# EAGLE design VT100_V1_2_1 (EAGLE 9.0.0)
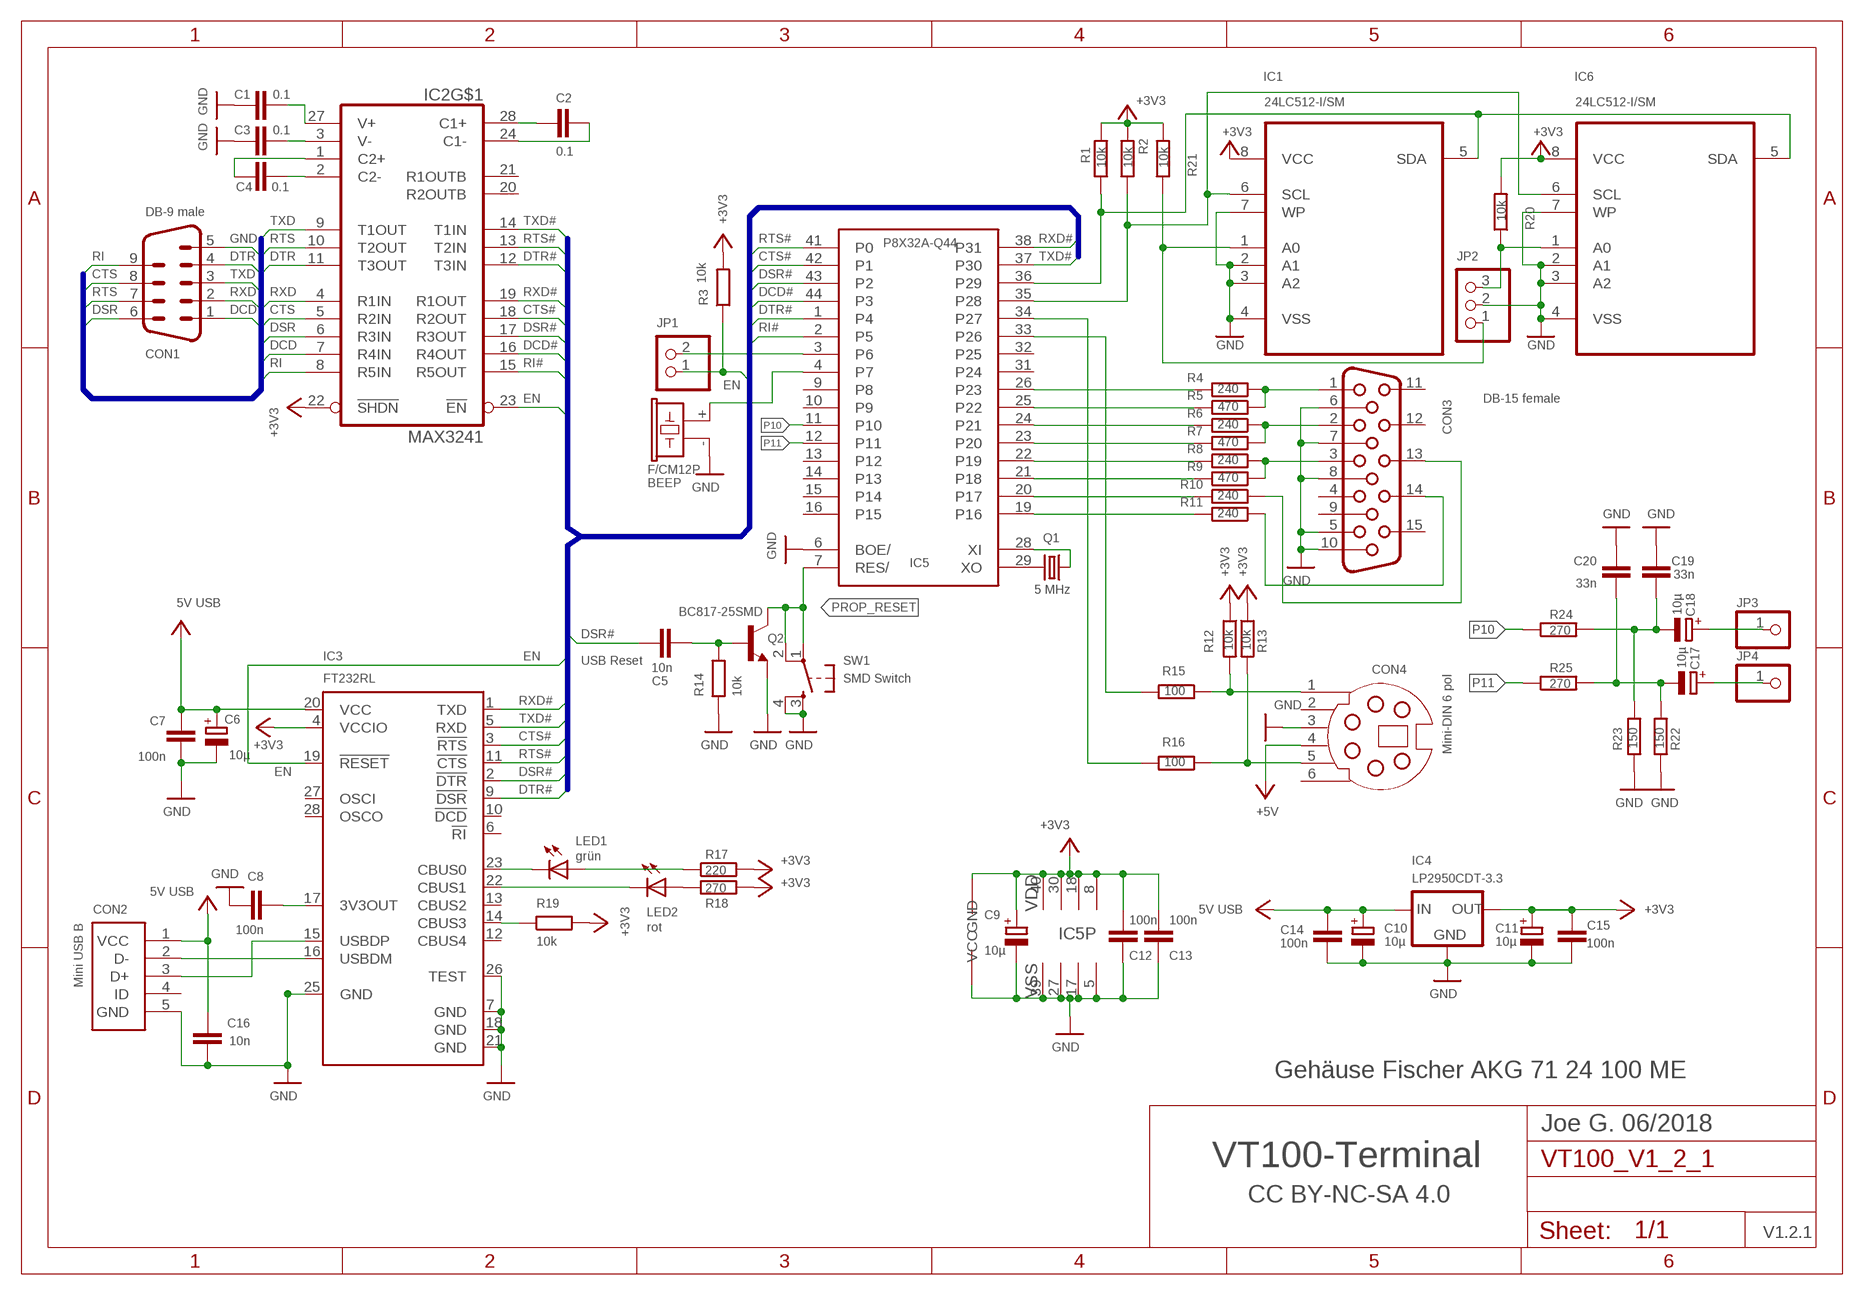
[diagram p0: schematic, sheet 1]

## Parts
BEEP  F/CM12P  [F/CM12P]
C1  0.1  C-EUC0805  [C0805]
C2  0.1  C-EUC0805  [C0805]
C3  0.1  C-EUC0805  [C0805]
C4  0.1  C-EUC0805  [C0805]
C5  10n  C-EUC0805  [C0805]
C6  10µ  CPOL-EUSMCC  [SMC_C]
C7  100n  C-EUC0805  [C0805]
C8  100n  C-EUC0805  [C0805]
C9  10µ  CPOL-EUSMCC  [SMC_C]
C10  10µ  CPOL-EUSMCC  [SMC_C]
C11  10µ  CPOL-EUSMCC  [SMC_C]
C12  100n  C-EUC0805  [C0805]
C13  100n  C-EUC0805  [C0805]
C14  100n  C-EUC0805  [C0805]
C15  100n  C-EUC0805  [C0805]
C16  10n  C-EUC0805  [C0805]
C17  10µ  CPOL-EUSMCC  [SMC_C]
C18  10µ  CPOL-EUSMCC  [SMC_C]
C19  33n  C-EUC0805  [C0805]
C20  33n  C-EUC0805  [C0805]
CON1  DB-9 male  M09-182  [182-009-MALE]
CON2  Mini USB B  65100516121  [65100516121]
CON3  DB-15 female  HF15H  [HDF15H]
CON4  Mini-DIN 6 pol  MDSSV-BC06  [SSV-BC06]
IC1  24LC512-I/SM  [SOIC127P794X203-8N]
IC2  MAX3241  [SSOP28]
IC3  FT232RL  [SSOP28]
IC4  LP2950CDT-3.3  [DPACK]
IC5  P8X32A-Q44  [P8X32A-Q44]
IC6  24LC512-I/SM  [SOIC127P794X203-8N]
JP1  PINHD-1X2  [1X02]
JP2  PINHD-1X3  [1X03]
JP3  PINHD-1X1  [1X01]
JP4  PINHD-1X1  [1X01]
LED1  grün  LEDSMT1206  [1206]
LED2  rot  LEDSMT1206  [1206]
Q1  5 MHz  CRYSTALHC49S  [HC49/S]
Q2  BC817-25SMD  [SOT23-BEC]
R1  10k  R-EU_M0805  [M0805]
R2  10k  R-EU_M0805  [M0805]
R3  10k  R-EU_M0805  [M0805]
R4  240  R-EU_R0805  [R0805]
R5  470  R-EU_R0805  [R0805]
R6  240  R-EU_R0805  [R0805]
R7  470  R-EU_R0805  [R0805]
R8  240  R-EU_R0805  [R0805]
R9  470  R-EU_R0805  [R0805]
R10  240  R-EU_R0805  [R0805]
R11  240  R-EU_M0805  [M0805]
R12  10k  R-EU_M0805  [M0805]
R13  10k  R-EU_M0805  [M0805]
R14  10k  R-EU_M0805  [M0805]
R15  100  R-EU_M0805  [M0805]
R16  100  R-EU_M0805  [M0805]
R17  220  R-EU_M0805  [M0805]
R18  270  R-EU_M0805  [M0805]
R19  10k  R-EU_M0805  [M0805]
R20  10k  R-EU_M0805  [M0805]
R21  10k  R-EU_M0805  [M0805]
R22  150  R-EU_M0805  [M0805]
R23  150  R-EU_M0805  [M0805]
R24  270  R-EU_M0805  [M0805]
R25  270  R-EU_M0805  [M0805]
SW1  SMD Switch  DTSM-6  [DTSM-6]

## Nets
+3V3: C9.+ C11.+ C12.2 C13.2 C15.2 IC1.8(VCC) IC2.22(!SHDN) IC2.26(VCC) IC3.4(VCCIO) IC4.3(OUT) IC5.8(VDD) IC5.18(VDD) IC5.30(VDD) IC5.40(VDD) IC6.8(VCC) R1.2 R2.2 R3.2 R12.1 R13.1 R17.2 R18.2 R19.2 R20.2 R21.2
+5V: C6.+ C7.2 C10.+ C14.2 C16.2 CON2.1(VCC) CON4.4 IC3.20(VCC) IC4.1(IN) ; supply symbol labelled 5V USB
CTS: CON1.8 IC2.5(R2IN)
CTS#: IC2.18(R2OUT) IC3.3(!RTS) IC5.42(P1)
DCD: CON1.1 IC2.7(R4IN)
DCD#: IC2.16(R4OUT) IC5.44(P3)
DM: CON2.2(D-) IC3.16(USBDM)
DP: CON2.3(D+) IC3.15(USBDP)
DSR: CON1.6 IC2.6(R3IN)
DSR#: C5.1 IC2.17(R3OUT) IC3.2(!DTR) IC5.43(P2)
DTR: CON1.4 IC2.11(T3OUT)
DTR#: IC2.12(T3IN) IC3.9(!DSR) IC5.1(P4)
EN: IC2.23(!EN) IC3.19(!RESET) JP1.1 R3.1
GND: BEEP.- C1.2 C3.1 C6.- C7.1 C8.1 C9.- C10.- C11.- C12.1 C13.1 C14.1 C15.1 C16.1 C19.2 C20.2 CON1.5 CON2.5(GND) CON3.5 CON3.6 CON3.7 CON3.8 CON3.10 CON4.3 IC1.2(A1) IC1.3(A2) IC1.4(VSS) IC1.7(WP) IC2.25(GND) IC3.7(GND) IC3.18(GND) IC3.21(GND) IC3.25(GND) IC3.26(TEST) IC4.4(GND) IC5.5(VSS) IC5.6(BOE/) IC5.17(VSS) IC5.27(VSS) IC5.39(VSS) IC6.2(A1) IC6.3(A2) IC6.4(VSS) IC6.7(WP) JP2.2 Q2.E R14.1 R22.2 R23.2 SW1.3 SW1.4
N$1: IC5.3(P6) JP1.2
N$2: BEEP.+ IC5.4(P7)
N$3: C4.2 IC2.2(C2-)
N$4: C5.2 Q2.B R14.2
N$5: IC5.29(XO) Q1.2
N$6: C4.1 IC2.1(C2+)
N$7: C3.2 IC2.3(V-)
N$8: IC3.23(CBUS0) LED1.C
N$9: IC3.22(CBUS1) LED2.C
N$10: LED2.A R18.1
N$11: C1.1 IC2.27(V+)
N$12: IC5.28(XI) Q1.1
N$13: C2.1 IC2.28(C1+)
N$14: C8.2 IC3.17(3V3OUT)
N$15: C2.2 IC2.24(C1-)
N$16: IC1.1(A0) JP2.1 R21.1
N$17: CON3.1 R4.1 R5.1
N$18: IC5.26(P23) R4.2
N$19: IC5.25(P22) R5.2
N$20: CON3.2 R6.1 R7.1
N$21: IC5.24(P21) R6.2
N$22: IC5.23(P20) R7.2
N$23: LED1.A R17.1
N$24: IC6.1(A0) JP2.3 R20.1
N$25: CON3.3 R8.1 R9.1
N$26: IC5.22(P19) R8.2
N$27: IC5.21(P18) R9.2
N$28: IC5.20(P17) R10.2
N$29: IC5.19(P16) R11.2
N$30: CON3.13 R10.1
N$31: CON3.14 R11.1
N$32: C17.- C20.1 R22.1 R25.2
N$33: C18.- C19.1 R23.1 R24.2
N$34: CON4.1 R12.2 R15.1
N$35: C18.+ JP3.1
N$36: CON4.5 R13.2 R16.1
N$37: C17.+ JP4.1
N$39: IC3.14(CBUS3) R19.1
P10: IC5.11(P10) R24.1
P11: IC5.12(P11) R25.1
P26: IC5.33(P26) R15.2
P27: IC5.34(P27) R16.2
PROP_RESET: IC5.7(RES/) Q2.C SW1.1 SW1.2
RI: CON1.9 IC2.8(R5IN)
RI#: IC2.15(R5OUT) IC5.2(P5)
RTS: CON1.7 IC2.10(T2OUT)
RTS#: IC2.13(T2IN) IC3.11(!CTS) IC5.41(P0)
RXD: CON1.2 IC2.4(R1IN)
RXD#: IC2.19(R1OUT) IC3.1(TXD) IC5.38(P31)
SCL: IC1.6(SCL) IC5.35(P28) IC6.6(SCL) R2.1
SDA: IC1.5(SDA) IC5.36(P29) IC6.5(SDA) R1.1
TXD: CON1.3 IC2.9(T1OUT)
TXD#: IC2.14(T1IN) IC3.5(RXD) IC5.37(P30)
Unconnected: CON2.4(ID) CON3.4 CON3.9 CON3.11 CON3.12 CON3.15 CON4.2 CON4.6 IC2.20(R2OUTB) IC2.21(R1OUTB) IC3.6(!RI) IC3.10(!DCD) IC3.12(CBUS4) IC3.13(CBUS2) IC3.27(OSCI) IC3.28(OSCO) IC5.9(P8) IC5.10(P9) IC5.13(P12) IC5.14(P13) IC5.15(P14) IC5.16(P15) IC5.31(P24) IC5.32(P25)

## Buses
DTE,DSR,DTR,RTS,CTS,TXD,RXD,RI,DCD,GND
TXD#,RXD#,RTS#,CTS#,DSR#,DCD#,DTR#,RI#,EN,DCD_U,RI_U

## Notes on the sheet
- USB Reset
- Gehäuse Fischer AKG 71 24 100 ME
- Joe G. 06/2018
- VT100-Terminal
- CC BY-NC-SA 4.0
- V1.2.1

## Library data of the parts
BEEP = buzzer:F/CM12P: BUZZER
C1-C5 C7 C8 C12-C16 C19 C20 = rcl:C-EU: CAPACITOR, European symbol
C6 C9-C11 C17 C18 = rcl:CPOL-EU: POLARIZED CAPACITOR, European symbol
CON1 = con-subd:M09: SUB-D; OC_FARNELL: unknown; OC_NEWARK: unknown
CON2 = Wuerth_Elektronik_eiCan_11_Communication_Connectors_2_4:65100516121: WR-COM SMT Horizontal 5 Contacts Mini USB Typ B
CON3 = con-subd:HF15: SUB-D; OC_FARNELL: unknown; OC_NEWARK: unknown
CON4 = con-yamaichi:MDSSV-BC06: YAMAICHI CONNECTOR; OC_FARNELL: unknown; OC_NEWARK: unknown
IC1 IC6 = 24LC512:24LC512-I/SM: 512K I2C Serial EEPROM; MPN: 24LC512-I/SM; OC_FARNELL: 9758038; OC_NEWARK: 62K0582; PACKAGE: SOIC-8; SUPPLIER: MICROCHIP
IC2 = Maxim_New:MAX3241: MAX3241
IC3 = ftdichip:FT232R: Source: http://www.ftdichip.com/Documents/DataSheets/DS_FT232R_v104.pdf
IC4 = v-reg:LP2950?*: Source: http://cache.national.com/ds/LP/LP2950.pdf
IC5 = parallax_propeller:P8X32A-Q44
JP1 = pinhead:PINHD-1X2: PIN HEADER
JP2 = pinhead:PINHD-1X3: PIN HEADER
JP3 JP4 = pinhead:PINHD-1X1: PIN HEADER
LED1 LED2 = led:LED: LED
Q1 = crystal:CRYSTAL: CRYSTAL; OC_FARNELL: 1667008; OC_NEWARK: unknown
Q2 = transistor-npn:BC817*: NPN Transistor
R1-R25 = rcl:R-EU_: RESISTOR, European symbol
SW1 = switch-tact:DTSM-6

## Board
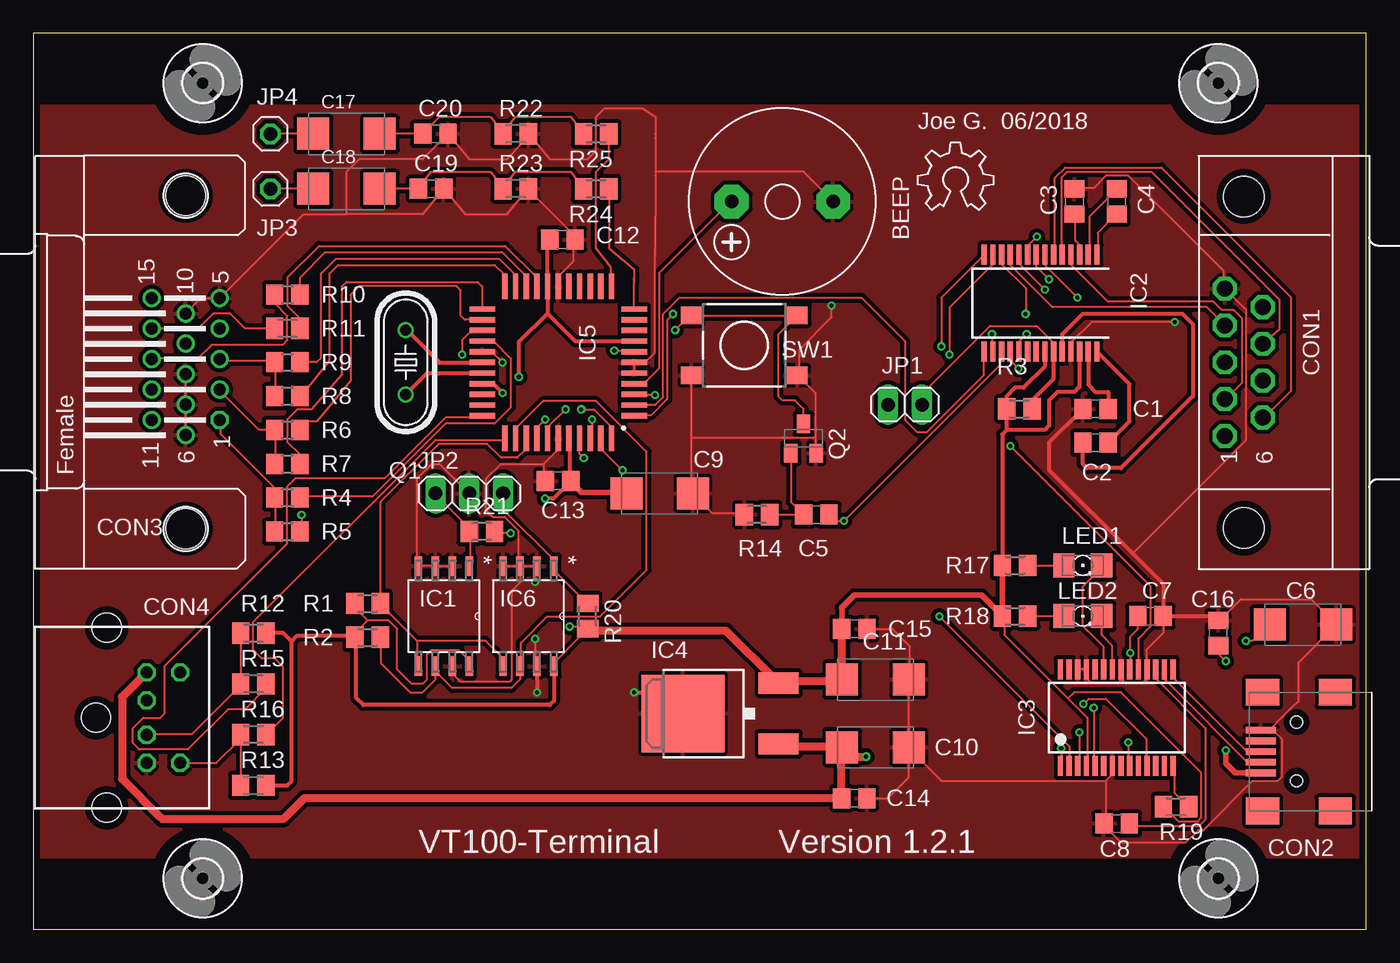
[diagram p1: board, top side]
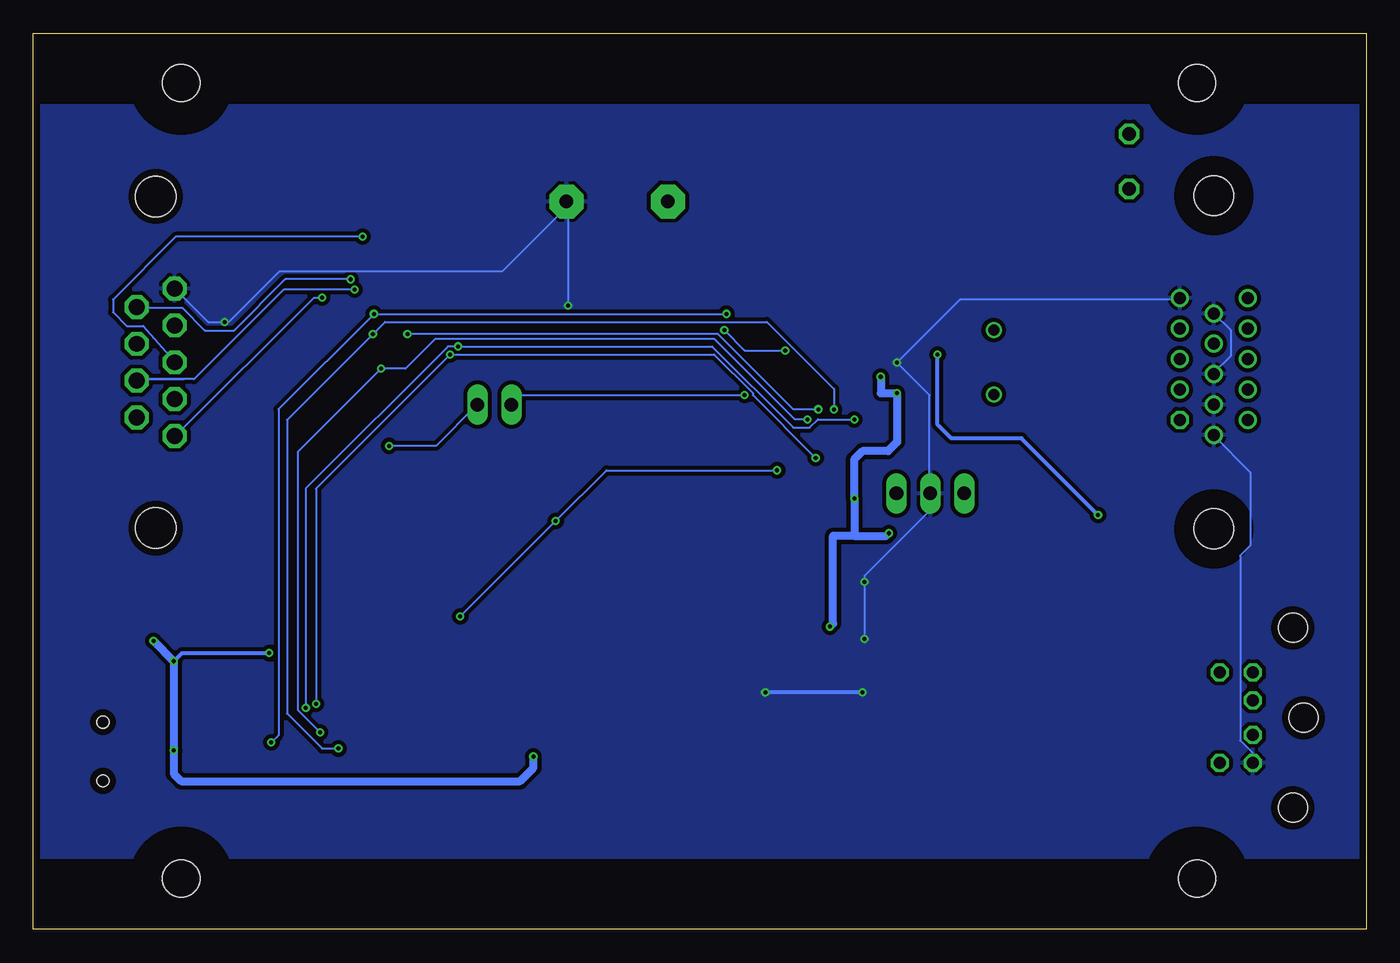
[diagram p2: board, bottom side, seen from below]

Size 100 x 67.23 mm. Coordinates in mm from the lower left corner, seen from the top.
Outline: 0,0 100,0 100,67.23 0,67.23 0,0
Copper layers (1*16): Top 0.035mm / dielectric 1.6mm / Bottom 0.035mm
Design rules "Elecrow_2-layer_PCB_eagle_rule": minimum track width 6mil, minimum drill 12mil, track to track 6mil, track to pad 6mil, pad to pad 6mil, via to via 8mil, smd to smd 0mil, copper to edge 20mil, drill to drill 10mil, minimum pad ring 6mil, minimum via ring 6mil, stop-mask expansion 0mil, vias tented up to drill 100mil, thermal gap 10mil
tRestrict: area 0,0 to 100,5; area 0,62.2 to 100,67.2
bRestrict: area 0,62.2 to 100,67.2; area 0,0 to 100,5

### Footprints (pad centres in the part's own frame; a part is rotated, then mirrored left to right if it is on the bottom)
F/CM12P = drill 1.016 pad 2.54 octagon: + 3.81,0; - -3.81,0
C0805 = smd 1.3 x 1.5: 1 -0.95,0; 2 0.95,0
SMC_C = smd 2.4 x 2.4: + -2.5,0; - 2.5,0
182-009-MALE = drill 1.194 pad 1.524 octagon: 1 -5.537,10.923; 2 -2.769,10.923; 3 0,10.923; 4 2.769,10.923; 5 5.537,10.923; 6 -4.153,8.08; 7 -1.384,8.08; 8 1.384,8.08; 9 4.153,8.08 | hole 3.048: -12.446,9.501; 12.446,9.501
65100516121 = smd 0.5 x 2.25: 1 -1.6,5.685; 2 -0.8,5.685; 3 0,5.685; 4 0.8,5.685; 5 1.6,5.685 | smd 2 x 2.5: Z1 -4.45,5.56; Z2 4.45,5.56; Z3 4.45,0.11; Z4 -4.45,0.11 | hole 0.9: -2.2,3.01; 2.2,3.01
HDF15H = drill 0.9 octagon: 1 4.329,2.54 | drill 0.9: 2 2.043,2.54; 3 -0.243,2.54; 4 -2.529,2.54; 5 -4.815,2.54; 6 5.472,0; 7 3.186,0; 8 0.9,0; 9 -1.386,0; 10 -3.672,0; 11 4.329,-2.54; 12 2.043,-2.54; 13 -0.243,-2.54; 14 -2.529,-2.54; 15 -4.815,-2.54 | hole 3: -12.5,0; 12.5,0
SSV-BC06 = drill 0.9 octagon: 1 1.3,8.5; 2 -1.3,8.5; 3 3.4,8.5; 4 -3.4,8.5; 5 3.4,11; 6 -3.4,11 | hole 2.2: -6.75,5.5; 0,4.7; 6.75,5.5
SOIC127P794X203-8N = smd 1.473 x 0.559: 1 -3.759,1.905; 2 -3.759,0.635; 3 -3.759,-0.635; 4 -3.759,-1.905; 5 3.759,-1.905; 6 3.759,-0.635; 7 3.759,0.635; 8 3.759,1.905
SSOP28 = smd 0.4 x 1.5: 1 -4.225,-3.625; 2 -3.575,-3.625; 3 -2.925,-3.625; 4 -2.275,-3.625; 5 -1.625,-3.625; 6 -0.975,-3.625; 7 -0.325,-3.625; 8 0.325,-3.625; 9 0.975,-3.625; 10 1.625,-3.625; 11 2.275,-3.625; 12 2.925,-3.625; 13 3.575,-3.625; 14 4.225,-3.625; 15 4.225,3.625; 16 3.575,3.625; 17 2.925,3.625; 18 2.275,3.625; 19 1.625,3.625; 20 0.975,3.625; 21 0.325,3.625; 22 -0.325,3.625; 23 -0.975,3.625; 24 -1.625,3.625; 25 -2.275,3.625; 26 -2.925,3.625; 27 -3.575,3.625; 28 -4.225,3.625
DPACK = smd 1.6 x 3: 1 -2.28,-4.8; 3 2.28,-4.8 | smd 5.8 x 6.2: 4 0,2.38
P8X32A-Q44 = smd 1.9 x 0.4: 1 -5.713,4.013; 2 -5.713,3.212; 3 -5.713,2.413; 4 -5.713,1.613; 5 -5.713,0.812; 6 -5.713,0.013; 7 -5.713,-0.787; 8 -5.713,-1.587; 9 -5.713,-2.388; 10 -5.713,-3.188; 11 -5.713,-3.987; 23 5.688,-3.987; 24 5.688,-3.188; 25 5.688,-2.388; 26 5.688,-1.587; 27 5.688,-0.787; 28 5.688,0.013; 29 5.688,0.812; 30 5.688,1.613; 31 5.688,2.413; 32 5.688,3.212; 33 5.688,4.013 | smd 0.4 x 1.9: 12 -4.013,-5.688; 13 -3.212,-5.688; 14 -2.413,-5.688; 15 -1.613,-5.688; 16 -0.812,-5.688; 17 -0.013,-5.688; 18 0.787,-5.688; 19 1.587,-5.688; 20 2.388,-5.688; 21 3.188,-5.688; 22 3.987,-5.688; 34 3.987,5.713; 35 3.188,5.713; 36 2.388,5.713; 37 1.587,5.713; 38 0.787,5.713; 39 -0.013,5.713; 40 -0.812,5.713; 41 -1.613,5.713; 42 -2.413,5.713; 43 -3.212,5.713; 44 -4.013,5.713
1X02 = drill 1.016 long: 1 -1.27,0; 2 1.27,0
1X03 = drill 1.016 long: 1 -2.54,0; 2 0,0; 3 2.54,0
1X01 = drill 1.016 octagon: 1 0,0
1206 = smd 1.6 x 1.803: A -1.422,0; C 1.422,0
HC49/S = drill 0.813: 1 -2.413,0; 2 2.413,0
SOT23-BEC = smd 1 x 1.4: B -0.95,-1.1; C 0,1.1; E 0.95,-1.1
M0805 = smd 1.3 x 1.6: 1 -0.95,0; 2 0.95,0
R0805 = smd 1.3 x 1.5: 1 -0.95,0; 2 0.95,0
DTSM-6 = smd 1.55 x 1.3: 1 -3.975,2.25; 2 3.975,2.25; 3 -3.975,-2.25; 4 3.975,-2.25
2,8 = hole 2.8: 0,0

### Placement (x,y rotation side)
BEEP  56.2,54.61 180 top
C1  79.69,39.05 180 top
C2  79.69,36.51 180 top
C3  78.11,54.61 270 top
C4  81.28,54.61 90 top
C5  58.74,31.11 180 top
C6  95.25,22.86 0 top
C7  83.82,23.5 180 top
C8  81.28,7.94 0 top
C9  46.99,32.7 0 top
C10  63.18,13.65 0 top
C11  63.18,18.73 0 top
C12  39.69,51.75 180 top
C13  39.37,33.66 0 top
C14  61.59,9.84 180 top
C15  61.59,22.54 180 top
C16  88.9,22.23 270 top
C17  23.5,59.69 0 top
C18  23.5,55.56 0 top
C19  29.84,55.56 0 top
C20  30.16,59.69 0 top
CON1  100.33,42.55 90 top
CON2  97.79,13.34 90 top
CON3  11.43,42.55 270 top
CON4  0,15.88 270 top
IC1  30.8,23.5 270 top
IC2  75.56,46.99 180 top
IC3  81.28,15.88 0 top
IC4  51.12,16.19 90 top
IC5  39.37,42.55 180 top
IC6  37.15,23.5 270 top
JP1  65.41,39.37 180 top
JP2  32.7,32.7 0 top
JP3  17.78,55.56 0 top
JP4  17.78,59.69 0 top
LED1  78.74,27.3 0 top
LED2  78.74,23.5 0 top
Q1  27.94,42.55 270 top
Q2  57.78,36.83 0 top
R1  25.08,24.45 180 top
R2  25.08,21.91 180 top
R3  73.98,39.05 180 top
R4  19.05,32.38 0 top
R5  19.05,29.84 0 top
R6  19.05,37.47 0 top
R7  19.05,34.92 0 top
R8  19.05,40.01 0 top
R9  19.05,42.55 0 top
R10  19.05,47.62 0 top
R11  19.05,45.09 0 top
R12  16.51,22.23 180 top
R13  16.51,10.79 180 top
R14  54.29,31.11 0 top
R15  16.51,18.41 0 top
R16  16.51,14.61 0 top
R17  73.66,27.3 180 top
R18  73.66,23.5 180 top
R19  85.72,9.21 180 top
R20  41.59,23.5 270 top
R21  33.66,29.84 0 top
R22  36.2,59.69 0 top
R23  36.2,55.56 0 top
R24  42.23,55.56 180 top
R25  42.23,59.69 180 top
SW1  53.34,43.81 0 top
U$1  [2,8]  12.7,63.5 0 top
U$3  [OSHW_6X200_NOTEXT]  66.36,53.98 0 top
U$4  [2,8]  88.9,63.5 0 top
U$5  [2,8]  88.9,3.81 0 top
U$6  [2,8]  12.7,3.81 0 top

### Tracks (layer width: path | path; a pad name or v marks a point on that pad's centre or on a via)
+3V3  (via drill 0.3)
  Top 0.152: C12.2 38.71,51.66 38.58,51.54 | 38.71,47.36 IC5.18 38.71,48.16 38.71,48.35 | 40.23,33.68 C13.2 | 40.23,36.73 IC5.40 | v35.81,29.72 34.75,29.72 R21.2 | 40.23,33.53 C13.2 | 34.59,40.84 33.83,40.84 IC5.30 | 44.35,32.77 C9.+ | 40.39,33.53 C13.2 | 17.53,10.82 R13.1 | 17.53,22.1 R12.1 | R2.2 24.23,21.95 24.32,22.04 24.32,22.42 25.08,23.18 | 24.23,24.08 24.23,24.38 R1.2 24.13,24.13 25.08,23.18 | 24.08,21.79 R2.2 | 41.45,22.4 41,21.95 | 41.45,22.4 R20.2 | 60.66,22.4 C15.2 60.66,22.55 | 60.66,18.75 C11.+ 60.66,18.59 | 55.93,18.59 IC4.3 55.78,18.59 | R20.2 41.6,22.4 41.45,22.4 | 78.49,42.67 78.49,43.28 IC2.26 | 77.64,17.31 72.85,22.1 72.85,23.47 R18.2 | 77.64,17.31 79.1,15.85 79.1,12.34 IC3.4 | 72.69,27.28 R17.2 72.69,27.43 | 72.69,23.62 R18.2 | R19.2 84.89,9.14 85.95,8.08 87.33,8.08 87.63,8.38 87.63,11.75 81.6,17.78 78.11,17.78 77.64,17.31 | 72.69,24.4 R18.2 | 24.23,21.79 R2.2 | 39.17,19.66 IC6.8 39.17,19.85 39.17,20.12 41,21.95 | 41,21.95 R20.2 | IC1.8 32.63,19.81 32.61,19.81 32.61,20.25 31.91,20.95 29.84,20.95 29.53,20.64 29.53,18.73 29.21,18.41 28.39,18.41 27.3,19.5 27.3,22.54 26.67,23.18 25.08,23.18 | v40.23,22.71 41.6,22.71 41.91,22.4 | 78.49,40.71 78.42,40.64 | 60.64,24.13 60.66,24.12
  Top 0.305: 40.23,36.73 40.23,33.68 | v38.41,32.31 39.01,32.31 40.23,33.53 | v35.2,40.23 34.59,40.84 | 72.69,27.43 72.69,37.13 73.03,37.47 | IC6.8 39.05,17.14 38.73,16.83 24.77,16.83 24.23,17.36 24.23,21.79 | R13.1 19.05,10.79 19.37,11.11 19.37,21.59 | 19.37,21.59 18.73,22.22 R12.1 | 19.37,21.59 19.81,22.04 24.32,22.04 | v36.42,41.45 36.42,44.04 38.58,46.2 | 78.42,40.64 78.11,40.32 76.83,40.32 76.2,39.69 76.2,37.78 75.88,37.47 73.03,37.47 | IC2.22 75.89,42.87 75.88,42.86 75.88,42.23 74.3,40.64 73.66,40.64 73.03,40.01 R3.2 73.03,37.47 | 38.58,51.54 IC5.18 38.58,46.2 | 38.58,46.2 40.65,44.13 IC5.8 | IC2.26 78.49,40.71
  Top 0.406: 44.35,32.77 41.15,32.77 40.39,33.53 | 72.69,23.62 72.69,24.4 72.69,27.28 | R18.2 71.12,25.09 61.6,25.09 60.64,24.13 | 60.66,24.12 60.66,22.4
  Top 0.61: 60.66,18.75 60.66,22.4 | 60.66,18.59 55.93,18.59 | 41.6,22.4 41.91,22.4 51.97,22.4 55.78,18.59
  Bottom 0.61: v36.42,41.45 36.42,40.23 v35.2,40.23 35.2,36.55 35.88,35.88 37.78,35.88 38.42,35.24 38.42,32.32 v38.41,32.31 38.41,29.54 38.42,29.53 | v40.23,22.71 40.01,22.94 40.01,29.53 38.42,29.53 | 38.42,29.53 36.01,29.53 v35.81,29.72
+5V  (via drill 0.3)
  Top 0.152: IC3.20 82.3,19.51 v82.3,20.73 82.3,21.97 82.87,22.55 C7.2 82.75,23.47 | v90.98,21.64 91.44,21.64 92.66,22.86 C6.+ | 89,21.18 C16.2 88.9,20.68 v89.46,20.12 | 90.98,11.89 92.05,11.89 CON2.1 | 60.5,9.91 C14.2 | 56.08,13.72 55.93,13.87 IC4.1 | 60.66,13.72 C10.+ 60.81,13.56 61,13.37 61.42,12.95 | 9.68,8.26 9.53,8.41
  Top 0.406: CON2.1 92.09,11.75 90.17,11.75 89.46,12.46 v89.46,13.41
  Top 0.61: 56.08,13.72 60.66,13.72 | 61.42,12.95 v62.48,12.95 | 61,13.37 60.65,13.02 C14.2 20.32,9.84 18.73,8.26 9.68,8.26 | CON4.4 6.67,17.44 6.67,11.27 9.53,8.41
  Bottom 0.305: v82.3,20.73 88.85,20.73 v89.46,20.12
  Bottom 0.61: v90.98,21.64 v89.46,20.12 v89.46,13.41 89.46,11.67 88.9,11.11 63.5,11.11 62.48,12.13 v62.48,12.95
CTS
  Top 0.152: IC2.5 77.11,50.75 77.11,56.39 77.57,56.84 83.88,56.84 93.47,47.26 93.47,45 CON1.8
CTS#  (via drill 0.3)
  Top 0.152: v78.49,14.78 78.49,12.34 IC3.3 | v73.91,42.06 73.3,42.67 73.3,43.28 IC2.18 | v41.91,38.25 41.91,36.88 IC5.42
  Bottom 0.152: v78.49,14.78 80.16,16.46 80.16,35.81 v73.91,42.06 | 73.76,42.06 v73.91,42.06 | v41.91,38.25 42.86,38.25 48.88,44.27 69.87,44.27 72.08,42.06 v73.91,42.06
DCD  (via drill 0.3)
  Top 0.152: v78.33,47.4 75.89,49.84 75.89,50.6 IC2.7
  Bottom 0.152: v78.33,47.4 78.94,47.4 89.31,37.03 CON1.1
DCD#  (via drill 0.3)
  Top 0.152: v71.93,44.65 71.93,43.43 IC2.16 | IC5.44 43.38,37.69 42.06,39.01 v41.11,39.01
  Bottom 0.152: v71.93,44.65 48.62,44.65 42.98,39.01 v41.11,39.01
DM
  Top 0.152: IC3.16 84.89,19.36 84.89,18.75 85.63,18 90.98,12.65 92.05,12.65 CON2.2
DP
  Top 0.152: IC3.15 85.65,19.36 85.65,18.75 90.98,13.41 92.05,13.41 CON2.3
DSR
  Top 0.152: IC2.6 76.66,50.75 76.66,56.39 77.42,57.15 84.63,57.15 94.37,47.41 94.37,40.42 92.99,39.04 CON1.6
DSR#  (via drill 0.3)
  Top 0.152: v67.97,23.47 77.72,13.72 77.72,12.34 IC3.2 | C5.1 59.74,31.09 60.2,30.63 v60.81,30.63 72.54,42.37 72.54,43.28 IC2.17 | v44.2,34.44 42.67,35.97 42.67,36.73 IC5.43
  Bottom 0.152: v67.97,23.47 v60.81,30.63 57,34.44 v44.2,34.44
DTR
  Top 0.152: IC2.11 73.3,50.6 73.3,49.84 76.33,46.81 76.35,46.79 76.47,46.67 88.05,46.67 CON1.4
DTR#  (via drill 0.3)
  Top 0.152: v82.14,14.02 82.14,12.34 IC3.9 | 72.69,49.84 72.69,50.6 IC2.12 72.64,49.91 74.45,48.1 v74.45,46.18 | v48.01,46.18 47.55,45.72 47.55,39.78 46.33,38.56 45.11,38.56 IC5.1
  Bottom 0.152: v48.01,46.18 v74.45,46.18 81.6,39.03 81.6,14.57 v82.14,14.02
EN  (via drill 0.3)
  Top 0.152: 76.5,42.67 76.5,43.28 IC2.23 76.5,43.43 76.5,44.04 75.29,45.26 71.78,45.26 66.75,40.23 66.75,39.47 JP1.1 | v73.3,36.27 83.82,25.76 83.82,22.71 82.91,21.79 IC3.19
  Top 0.305: IC2.23 76.52,43.34 76.52,41.27 74.93,39.69 R3.1
  Bottom 0.152: v73.3,36.27 69.8,36.27 66.75,39.32 JP1.1
GND  (via drill 0.3)
  Top 0.152: 65.53,18.75 C11.- | 80.47,11.12 80.47,8.08 C8.1 | 80.47,11.12 80.92,11.58 80.92,12.19 IC3.7 | 62.64,9.91 C14.1 64.14,9.84 65.68,11.39 65.68,13.72 | 65.53,13.56 C10.- | 80.47,11.12 68.12,11.12 65.68,13.56 C10.- | 65.68,13.72 65.68,18.59 C11.- | 65.68,13.72 C10.- | 50.9,16.15 48.77,16.15 IC4.4 | v85.65,45.57 79.4,45.57 77.88,44.04 77.88,43.43 IC2.25 | C3.1 78.18,55.63 79.55,55.63 80.47,56.54 82.14,56.54 89.31,49.38 89.31,48.16 CON1.5 | IC3.26 78.49,19.51 78.94,19.51 IC3.25 79.1,19.36 79.1,18.75 79.4,18.44 81.38,18.44 81.69,18.75 | 81.69,18.75 81.69,19.36 IC3.21 | 81.69,18.75 81.99,18.44 83.21,18.44 83.52,18.75 83.52,19.36 IC3.18 | 84.89,23.47 85.04,23.47 C7.1 | 88.7,23.47 88.85,23.32 C16.1 89,23.16 90.6,24.77 95.89,24.77 97.75,22.9 C6.- 94.93,20.04 94.93,17.14 94.36,16.57 94.35,16.57 93.75,15.96 92.72,14.94 CON2.5 | 84.89,23.47 C7.1 | 92.05,14.94 CON2.5 | 83.67,19.51 IC3.18 | 89.46,48.01 CON1.5 | 80.47,7.92 C8.1 | 92.2,14.78 CON2.5 | 58.67,36.88 58.67,40.23 57.45,41.45 SW1.4 | 58.67,36.88 58.67,35.81 Q2.E | 49.38,36.88 49.38,32.77 C9.- 49.53,32.61 50.9,31.24 53.34,31.24 R14.1 | 49.38,36.88 49.38,41.45 SW1.3 | 49.38,36.88 58.67,36.88 | 45.11,41.76 IC5.5 IC5.6 | 45.11,42.52 IC5.6 | 46.63,50.48 46.63,43.28 45.88,42.53 IC5.6 | 46.63,50.48 46.63,51.05 | 59.05,55.56 59.89,54.71 BEEP.- | 59.05,55.56 58.37,56.24 | 57.45,41.6 SW1.4 | 38.28,34.92 39.32,35.97 39.32,36.73 IC5.39 | 38.56,33.68 C13.1 38.28,33.8 38.28,34.92 | IC1.7 31.55,19.66 31.55,19.09 32.07,18.57 35.72,18.57 35.88,18.73 35.88,25.4 36.51,26.04 IC6.3 | 35.36,27.13 IC6.4 IC6.3 | 36.42,27.13 IC6.3 | IC6.3 36.58,27.28 37.64,27.28 IC6.2 37.64,27.13 v37.64,26.06
  Top 0.152: IC6.3 36.42,27.28 36.42,29.87 35.36,30.94 34.47,30.94 33.97,31.43 33.97,33.81 35.09,34.92 38.28,34.92 | 28.96,27.28 30.02,27.28 IC1.3 30.18,27.28 31.39,27.28 IC1.2 | 28.8,27.28 28.96,27.28 | 28.96,27.28 IC1.4 28.8,27.28 | v37.64,21.79 37.64,19.81 IC6.7 | v35.2,42.52 34.44,43.28 33.83,43.28 IC5.27 | 28.8,27.28 28.8,33.83 29.9,34.92 30.48,34.92 30.48,34.9 32.61,32.77 JP2.2 | 31.24,59.59 C20.2 | 37.03,59.59 R22.2 | IC5.17 39.47,48.31 39.47,49.07 40.54,50.14 40.54,51.66 C12.1 40.54,51.82 40.54,52.12 37.19,55.47 R23.2 | 30.94,55.47 C19.2 | C19.2 | 37.03,55.47 R23.2 | 31.09,59.59 C20.2 | 30.79,55.47 C19.2 | 13.87,47.24 CON3.5 | CON3.6 CON3.7 CON3.8 | 14.02,47.4 CON3.5 | R22.2 37.19,59.59 35.56,57.78 32.7,57.78 C20.2 | CON1.5 90.98,46.51 90.98,36.69 82.48,28.19 | 84.77,23.58 84.89,23.47 | CON3.5 20.27,53.66 23.5,53.66 | 30.8,55.4 C19.2 | 23.5,53.66 23.5,56.83 24.45,57.78 29.21,57.78 C20.2 | 31.11,59.37 C20.2 | SW1.4 57.47,41.72 57.47,43.5 59.89,45.92 v59.89,46.79 | CON3.10 12.57,47.36 CON3.5 | CON2.5 93.02,14.94 93.66,14.29 93.66,11.43 93.36,11.12 91.45,11.12 87.77,7.44 87.39,7.44 86.46,6.51 81.6,6.51 80.33,7.78 C8.1 | 62.55,21.87 C15.1 64.45,22.54 65.72,21.27 65.72,18.77 C11.- | C7.1 84.77,22.22 83.5,20.95 83.5,19.55 IC3.18 | C19.2 32.38,53.66 35.56,53.66 R23.2 | C19.2 29.21,53.66 23.5,53.66 | 59.05,55.56 57.78,56.83 46.67,56.83 46.67,56.52 | 46.67,56.52 46.63,50.48 | 46.67,59.69 46.67,59.37 | 46.67,59.37 46.67,56.52 | R22.2 38.73,57.78 41.59,57.78 42.23,58.42 42.23,60.96 42.86,61.59 45.72,61.59 46.67,60.96 46.67,59.37
  Top 0.305: 88.7,23.47 85.04,23.47 | IC6.7 v37.78,17.78 | v45.09,17.78 46.04,17.78 48.77,16.15 | C1.2 76.2,36.51 76.2,34.47 82.48,28.19 84.77,25.89 84.77,23.58
  Bottom 0.152: CON1.5 89.31,48.01 86.87,45.57 v85.65,45.57 85.34,45.57 81.53,49.38 64.81,49.38 59.89,54.29 | 59.89,54.29 59.89,54.56 BEEP.- | 59.89,54.29 v59.89,46.79 | v37.64,21.79 v37.64,26.06 37.64,26.52 32.77,31.39 32.77,32.61 JP2.2 32.77,32.77 32.77,40.08 v35.2,42.52 30.48,47.24 14.02,47.24 CON3.5 | CON4.3 8.53,12.5 8.53,13.26 9.45,14.17 9.45,28.04 8.69,28.8 8.69,34.29 11.43,37.03 CON3.6 | CON3.8 11.43,41.76 10.16,43.03 | CON3.10 10.16,44.95 10.16,43.03 | 10.16,43.03 10.16,43.02
  Bottom 0.305: v37.78,17.78 v45.09,17.78
  pour Top (isolate 0.305): 0,67.31 100.01,67.31 100.01,0 0,0
  pour Bottom (isolate 0.305): 0,66.99 100.01,66.99 100.01,0 0,0
N$1  (via drill 0.3)
  Top 0.152: v46.63,40.08 45.11,40.08 IC5.3
  Bottom 0.152: v46.63,40.08 63.4,40.08 64.01,39.47 JP1.2
N$2
  Top 0.152: IC5.4 45.11,41 45.87,41 46.94,42.06 46.94,49.23 52.27,54.56 BEEP.+
N$3
  Top 0.152: IC2.2 79.25,50.75 79.25,53.49 81.23,55.47 C4.2
N$4
  Top 0.152: 56.84,35.66 Q2.B 56.84,32.07 C5.2 | 55.32,31.24 R14.2 C5.2 | C5.2
N$5
  Top 0.152: 33.68,41.6 IC5.29
  Top 0.305: Q1.2 29.54,41.73 IC5.29
N$6
  Top 0.152: IC2.1 79.86,50.75 79.86,52.27 81.23,53.65 C4.1
N$7
  Top 0.152: C3.2 78.18,53.65 78.18,51.66 78.49,51.36 78.49,50.75 IC2.3
N$8
  Top 0.152: LED1.C 80.01,27.28 80.01,26.99 78.74,25.72 78.74,22.76 79.1,22.4 79.17,22.33 80.31,21.19 IC3.23
N$9
  Top 0.152: 80.92,19.51 IC3.22 80.95,21.28 80.16,22.07 LED2.C | 80.16,23.47 LED2.C | LED2.C
N$10
  Top 0.152: R18.1 74.68,23.47 77.27,23.47 LED2.A
N$11
  Top 0.305: IC2.27 79.14,40.88 79.69,40.32 80.64,40.32 C1.1
N$12
  Top 0.152: IC5.28 | 28.04,44.96 Q1.1
  Top 0.305: IC5.28 30.48,42.52 28.04,44.96
N$13
  Top 0.152: 79.86,43.28 IC2.28
  Top 0.305: C2.1 82.23,38.1 82.23,40.91 79.86,43.28
N$14
  Top 0.152: 82.3,7.92 C8.2 82.39,7.77 87.48,7.77 87.94,8.23 87.94,15.09 84.28,18.75 84.28,19.36 IC3.17
N$15
  Top 0.152: 77.27,43.43 IC2.24
  Top 0.305: C2.2 78.74,34.92 79.06,34.61 81.6,34.61 86.26,39.27 87,40.01 87,45.4 86.2,46.2 78.74,46.2 77.19,44.65 IC2.24
N$16
  Top 0.152: IC1.1 32.77,27.28 32.77,29.72 R21.1 32.61,29.87 32.61,30.18 30.18,32.61 JP2.1
N$17
  Top 0.152: R5.1 18.14,29.87 18.14,32.31 R4.1 17.98,32.46 17.98,33.22 14.02,37.19 14.02,38.1 CON3.1
N$18
  Top 0.152: R4.2 20.12,32.46 25.45,32.46 30.94,37.95 34.59,37.95 35.81,39.17 35.81,42.82 34.59,44.04 33.83,44.04 IC5.26
N$19  (via drill 0.3)
  Top 0.152: v20.12,31.09 20.12,29.87 R5.2 | v32.16,43.13 32.16,44.2 32.77,44.81 33.68,44.81 IC5.25
  Bottom 0.305: v20.12,31.09 25.86,36.83 31.11,36.83 32.16,37.87 v32.16,43.13
N$20
  Top 0.152: R7.1 18.14,35.05 18.14,37.34 R6.1 17.98,37.49 16.92,37.49 14.02,40.39 CON3.2
N$21
  Top 0.152: R6.2 20.12,37.49 20.12,37.8 20.42,38.1 21.27,38.1 23.8,41.16 23.8,47.61 24.45,48.26 31.75,48.26 32.07,47.94 32.07,46.04 32.37,45.73 IC5.24
N$22
  Top 0.152: R7.2 19.96,35.05 19.96,35.66 19.05,36.58 19.05,38.25 19.81,39.01 20.88,39.01 23.18,41.63 23.18,48.26 23.5,48.58 33.34,48.58 33.68,48.23 IC5.23 33.68,46.48
N$23
  Top 0.152: R17.1 74.68,27.28 77.27,27.28 LED1.A
N$24
  Top 0.152: R20.1 41.45,24.54 39.17,26.82 39.17,27.13 IC6.1 39.01,27.28 39.01,27.74 35.36,31.39 35.36,32.61 JP2.3
N$25
  Top 0.152: R8.1 18.14,40.08 18.14,42.52 R9.1 17.98,42.67 14.02,42.67 CON3.3
N$26
  Top 0.152: 22.15,42.62 22.14,42.61 | 22.14,42.61 20.12,40.08 R8.2 | 22.14,42.61 22.23,42.7 22.23,49.21 22.86,49.85 34.61,49.85 35.38,49.07 IC5.22
N$27
  Top 0.152: 36.12,49.07 36.12,48.31 36.17,48.24 | 36.17,48.24 IC5.21 | R9.2 21.27,42.55 21.59,42.86 21.59,49.21 22.7,50.32 34.92,50.32 36.17,49.08 36.17,48.24
N$28
  Top 0.152: R10.2 20.12,47.7 | R10.2 20,48.89 21.91,50.8 35.15,50.8 36.88,49.07 36.88,48.31 IC5.20 | 19.68,48.12 19.68,47.94 R10.2
N$29
  Top 0.152: 37.64,49.05 37.64,49.07 | R11.2 19.96,45.11 19.96,45.87 19.05,46.79 19.05,48.9 21.43,51.28 35.41,51.28 37.64,49.05 | IC5.19 37.64,49.05
N$30
  Top 0.152: R10.1 18.14,47.55 18.14,46.94 19.05,46.02 19.05,44.2 18.7,43.85 13.37,43.85 12.34,42.82 8.99,42.82 CON3.13
N$31
  Top 0.152: 17.98,45.11 R11.1 15.88,45.09 14.76,46.2 13.49,46.2 12.38,45.09 8.9,45.09 | 8.9,45.09 CON3.14 | CON3.14 8.9,45.09
N$32
  Top 0.152: C20.1 29.11,59.74 26.06,59.74 C17.- | 35.36,59.74 R22.1 | 41.15,59.74 R25.2 | R25.2 | 29.26,59.74 C20.1 | R22.1 35.2,59.74 34.29,60.96 30.48,60.96 C20.1 | R22.1 36.2,60.96 40.32,60.96 R25.2
N$33
  Top 0.152: C19.1 28.8,55.63 26.06,55.63 C18.- | 35.36,55.63 R23.1 | 41.15,55.63 R24.2 40.32,56.83 36.2,56.83 R23.1 | 28.96,55.63 C19.1 | R23.1 35.2,55.63 34.29,56.83 29.84,56.83 C19.1
N$34
  Top 0.152: R12.2 15.54,22.1 15.54,18.44 R15.1 15.54,18.29 11.89,14.63 8.53,14.63 CON4.1
N$35
  Top 0.152: C18.+ 20.88,55.63 17.83,55.63 JP3.1
N$36
  Top 0.152: 15.54,14.29 15.54,14.48 R16.1 | 15.54,14.29 15.54,10.82 R13.2 | CON4.5 13.73,12.47 15.54,14.29
N$37
  Top 0.152: C17.+ 20.88,59.74 17.83,59.74 JP4.1
N$39
  Top 0.152: IC3.14 85.65,12.19 85.65,10.21 86.56,9.3 R19.1
P10
  Top 0.152: 43.28,55.47 R24.1 | R24.1 | R24.1 43.18,51.12 45.09,49.53 45.09,48.58 | IC5.11 45.09,48.58 | 45.09,48.58 45.09,48.9
P11
  Top 0.152: 43.13,59.59 R25.1 43.18,57.78 42.23,56.83 42.23,51.12 43.34,49.69 IC5.12 43.28,48.31
P26
  Top 0.152: 17.37,18.29 R15.2 17.46,18.09 15.88,16.51 14.61,16.51 11.59,13.49 7.94,13.49 7.46,13.97 7.46,15.08 8.26,15.88 9.53,15.88 9.84,16.19 9.84,19.75 19.05,28.96 19.05,33.22 19.66,33.83 26.36,33.83 30.94,38.41 33.68,38.41 IC5.33
P27
  Top 0.152: 17.53,14.63 R16.2 18.73,15.88 18.73,19.68 18.1,20.32 17.14,20.32 16.51,20.95 16.51,23.06 30.18,36.73 35.36,36.73 IC5.34
PROP_RESET  (via drill 0.3)
  Top 0.152: 57.76,37.95 Q2.C 57.78,39.05 57.15,39.69 56.2,39.69 55.88,40.01 55.88,44.63 SW1.2 57.3,46.02 57.26,46.06 SW1.1 | 49.38,46.02 SW1.1 | v43.59,43.43 44.96,43.43 IC5.7 | v48.16,44.96 49.23,46.02 SW1.1
  Bottom 0.152: v43.59,43.43 46.63,43.43 v48.16,44.96
RI  (via drill 0.3)
  Top 0.152: 75.29,50.6 IC2.8 75.24,49.73 v76.2,48.77
  Bottom 0.152: CON1.9 92.2,46.63 88.84,46.63 87.13,44.93 84.93,44.93 81.09,48.77 v76.2,48.77
RI#
  Top 0.152: IC2.15 71.32,42.96 71.32,41.59 67.06,37.33 66.29,37.33 65.39,38.23 65.39,44.12 65.41,44.13 62.14,47.4 48.46,47.4 47.24,46.18 47.24,39.93 47,39.68 46.79,39.47 46.65,39.33 IC5.2
RTS  (via drill 0.3)
  Top 0.152: v75.89,48.01 74.07,49.84 74.07,50.6 IC2.10
  Bottom 0.152: 92.2,41.3 88.7,41.3 | 92.2,41.3 CON1.7 | v75.89,48.01 81.22,48.01 87.95,41.27 92.18,41.27 92.2,41.3
RTS#  (via drill 0.3)
  Top 0.152: v68.73,43.13 68.73,46.63 71.93,49.84 71.93,50.6 IC2.13 | 83.52,12.34 IC3.11 83.5,12.3 83.5,14.29 80.49,17.3 79.18,17.3 v78.79,16.92 | v41.3,35.36 41,35.66 41,36.73 IC5.41
  Bottom 0.152: v78.79,16.92 78.79,33.07 v68.73,43.13 48.92,43.13 46.02,40.23 46.02,40.08 v41.3,35.36
RXD
  Top 0.152: IC2.4 77.88,50.6 77.88,49.84 80.62,47.09 88.53,47.09 89.14,46.48 90.04,46.48 90.68,45.85 90.68,41 89.46,39.78 CON1.2
RXD#  (via drill 0.3)
  Top 0.152: v77.11,13.56 77.11,12.34 IC3.1 | 74.07,43.43 IC2.19 | v39.93,39.01 38.71,37.8 38.71,36.88 IC5.38 | 73.98,43.4 73.98,44.13 74.5,44.65 v74.52,44.65
  Top 0.305: 73.98,43.4 IC2.19
  Bottom 0.152: v39.93,39.01 39.93,40.54 44.96,45.57 73.61,45.57 v74.52,44.65 80.96,38.21 80.96,16.19 78.33,13.56 v77.11,13.56
SCL
  Top 0.152: 30.02,19.66 IC1.6 30.16,19.37 | R2.1 26.06,21.79 26.06,19.98 28.26,17.78 29.21,17.78 30.16,18.73 30.16,19.37 | 36.42,19.66 IC6.6 | IC5.35 36.27,36.88 36.27,37.64 38.25,39.62 42.22,39.62 46.02,35.81 46.02,26.98 42.52,23.47 38.56,23.47 36.58,21.49 36.58,19.81 IC6.6 | IC6.6 36.51,18.73 35.88,18.1 31.43,18.1 30.16,19.37
SDA
  Top 0.152: 28.8,21.64 28.8,19.81 IC1.5 | 28.8,21.64 26.06,24.38 R1.1 26.03,32.06 30.39,36.42 34.06,36.42 35.1,35.38 36.3,35.38 36.88,35.97 36.88,36.73 IC5.36 | IC6.5 35.24,20.32 33.92,21.64 28.8,21.64
TXD  (via drill 0.3)
  Top 0.152: v75.29,51.97 74.68,51.36 74.68,50.75 IC2.9
  Bottom 0.152: CON1.3 89.46,42.67 91.75,45.28 92.99,45.28 94.02,46.3 94.02,47.27 89.32,51.97 v75.29,51.97
TXD#  (via drill 0.3)
  Top 0.152: v79.55,16.61 79.55,12.34 IC3.5 | v68.12,43.74 68.12,47.4 71.32,50.6 IC2.14 | v38.41,38.25 37.8,37.64 37.8,36.88 IC5.37
  Bottom 0.152: v79.55,16.61 79.55,33.07 68.89,43.74 v68.12,43.74 49.07,43.74 42.98,37.64 41.76,37.64 41.15,38.25 v38.41,38.25

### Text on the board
tNames: Joe G. 06/2018 | VT100-Terminal | Version 1.2.1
